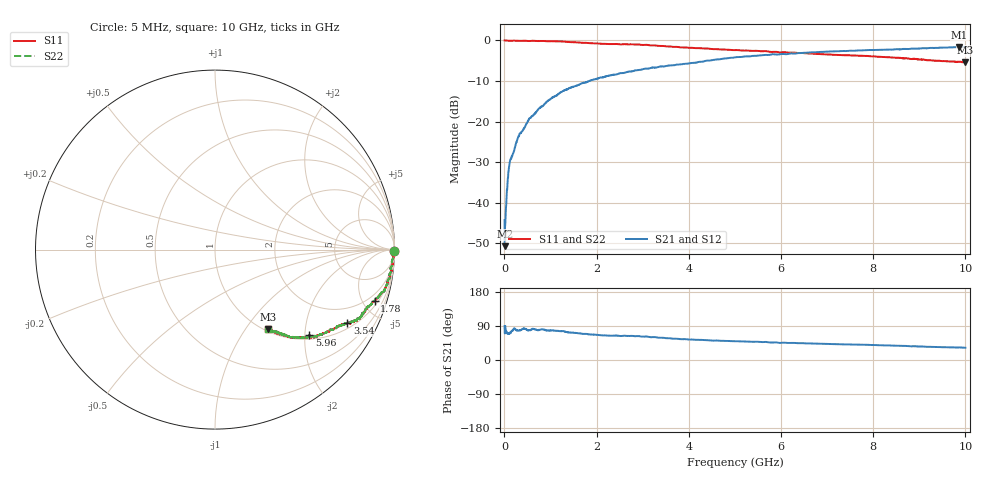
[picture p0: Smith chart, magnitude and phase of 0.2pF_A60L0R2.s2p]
! Amotech Co.,Ltd.
! http://www.amotech.co.kr/
! Part Number: A60L0R2
! These Parameters are Measured in Series Mode Connection
! Operation Temp=25[degC], DC Bias Voltage=0[V]
! Freq. Start=5[MHz] Stop=10[GHz], 2000[Steps]
! Date: Monday, July 14, 2020, 09:24:13
# GHZ S RI R 50.000000
!Freq.(Hz) S11(Real) S11(Imag) S21(Real) S21(Imag) S12(Real) S12(Imag) S22(Real) S22(Imag)
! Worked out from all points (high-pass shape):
!   2000 points, 5 MHz to 10 GHz, reference 50 ohm
!   highest |S21| = -1.59 dB at 9.865 GHz (marker M1); lowest = -50.7 dB at 10 MHz (marker M2)
!   |S21| within 3 dB of the highest: 4.692 GHz to end of sweep
!   lowest |S11| = -5.4 dB at 10 GHz (marker M3), VSWR 3.30, Z = 51.7 - j64.4 ohm
!   |S11| at or under -10 dB: nowhere
!   |S22| runs from -5.4 to 0.0 dB; largest |S21 - S12| = 1.4e-15
!   S11 on the Smith chart (normalised r, x): 5 MHz: open; 1.78 GHz: 1.38, -6.11; 3.54 GHz: 1.21, -3.45; 5.96 GHz: 1.09, -2.11; 10 GHz: 1.03, -1.29
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0.005  1 -0.00608  4.46e-05 0.00608  4.46e-05 0.00608  1 -0.00608
0.01  0.999 -0.00274  0.000983 0.00274  0.000983 0.00274  0.999 -0.00274
0.045  0.9971 -0.0106  0.0029 0.0106  0.0029 0.0106  0.9971 -0.0106
0.09  0.9913 -0.0225  0.00865 0.0225  0.00865 0.0225  0.9913 -0.0225
0.125  0.9895 -0.0314  0.0105 0.0314  0.0105 0.0314  0.9895 -0.0314
0.15  0.9909 -0.0339  0.00914 0.0339  0.00914 0.0339  0.9909 -0.0339
0.275  0.9877 -0.0577  0.0123 0.0577  0.0123 0.0577  0.9877 -0.0577
0.335  0.9858 -0.0697  0.0142 0.0697  0.0142 0.0697  0.9858 -0.0697
0.555  0.978 -0.1087  0.022 0.1087  0.022 0.1087  0.978 -0.1087
0.935  0.9636 -0.1749  0.0364 0.1749  0.0364 0.1749  0.9636 -0.1749
1.275  0.9439 -0.2315  0.0561 0.2315  0.0561 0.2315  0.9439 -0.2315
1.675  0.8965 -0.2769  0.1035 0.2769  0.1035 0.2769  0.8965 -0.2769
1.78  0.8891 -0.2843  0.1109 0.2843  0.1109 0.2843  0.8891 -0.2843
2.25  0.8414 -0.33  0.1586 0.33  0.1586 0.33  0.8414 -0.33
3.34  0.7572 -0.4026  0.2428 0.4026  0.2428 0.4026  0.7572 -0.4026
3.54  0.7373 -0.411  0.2627 0.411  0.2627 0.411  0.7373 -0.411
5.005  0.5967 -0.4702  0.4033 0.4702  0.4033 0.4702  0.5967 -0.4702
5.96  0.525 -0.4779  0.475 0.4779  0.475 0.4779  0.525 -0.4779
6.67  0.4826 -0.4926  0.5174 0.4926  0.5174 0.4926  0.4826 -0.4926
8.335  0.394 -0.4807  0.606 0.4807  0.606 0.4807  0.394 -0.4807
9.865  0.303 -0.4548  0.697 0.4548  0.697 0.4548  0.303 -0.4548
10  0.2979 -0.4442  0.7021 0.4442  0.7021 0.4442  0.2979 -0.4442
